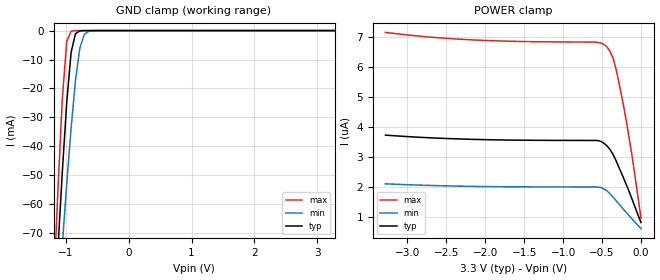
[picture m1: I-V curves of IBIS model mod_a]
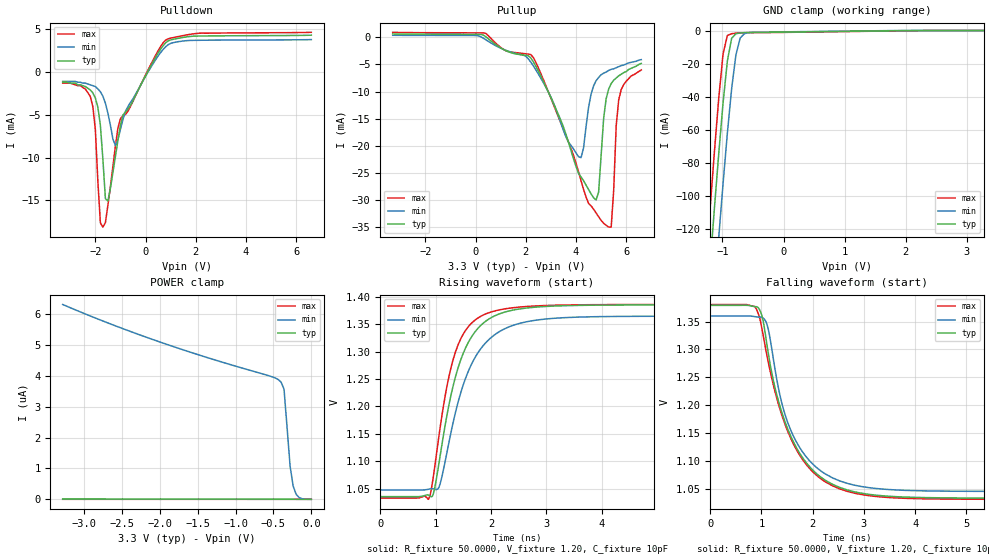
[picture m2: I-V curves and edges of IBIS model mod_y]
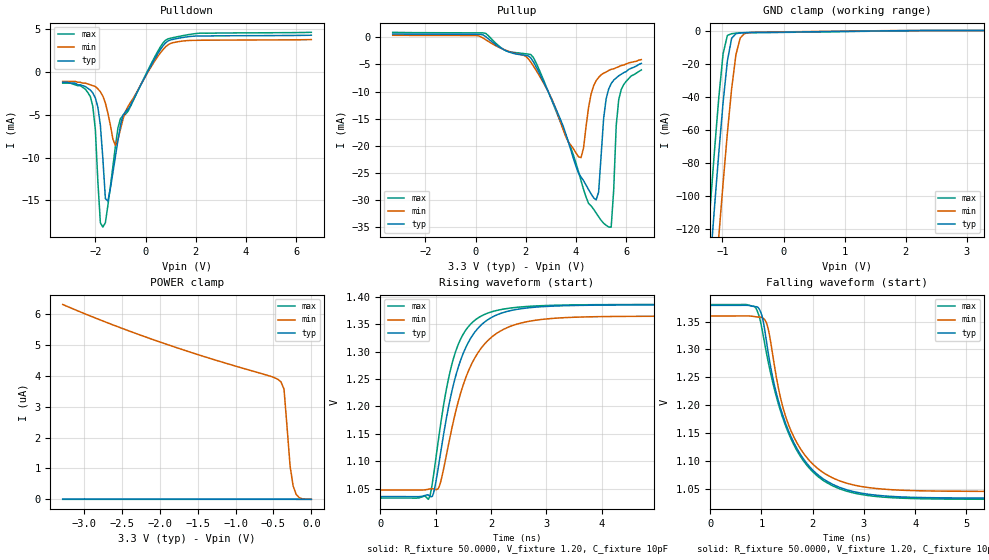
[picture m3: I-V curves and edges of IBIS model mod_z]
| IBIS (I/O, Buffer, Information, Specification) Model, officially
| electronic behavioral standard for Buffer structures of digital pins.
[IBIS ver]  4.0
[File name] rhflvds31a_3v3_rev3.ibs
[File Rev]  1.0
[Date]   28 Apr 2021
[Source]   CAD & Design Services (Catania) - STMicroelectronics
[Notes]
   (Note1)  This IBIS model is the model of the product with package
   (Flat16 package elements);
   (Note2)  This IBIS model is extracted with nominal 3.3V power supply
   (min:3.0V, typ:3.3V, max:3.6V);
   (Note3)  This IBIS model has some Notes about the non-monotonicity
   of the I-V curves, but they are not indicative of problems
   inside the model;
[Disclaimer] Customers are solely responsible for all aspects of their
   own product designs or applications using this IBIS Model.
   STMicroelectronics assumes no liability for Custmer
   Designs and applications associated to this IBIS Model.
   In the use of this IBIS Model Customer shall not modify,
   disassemble, alter this Model in whole or in part.
   If Customers do not accept these terms, the IBIS Model
   may not be used. For any problems or modifications please
   contact STMicroelectronics (www.st.com).
[Copyright] (c) 2021 STMicroelectronics
|   Component RHFLVDS31A
[Component] RHFLVDS31A
[Manufacturer] STMicroelectronics
[Package]
| variable   typ   min   max
R_pkg   0.0   0.0   0.0
L_pkg   0.0H   0.0H   0.0H
C_pkg   0.0F   0.0F   0.0F
[Pin]   signal_name   model_name   R_pin   L_pin   C_pin
1   1A   mod_a   0.0   0.0   0.0
2   1Y   mod_y   0.0   0.0   0.0
3   1Z   mod_z   0.0   0.0   0.0
4   G   mod_g   0.0   0.0   0.0
5   2Z   mod_z   0.0   0.0   0.0
6   2Y   mod_y   0.0   0.0   0.0
7   2A   mod_a   0.0   0.0   0.0
8   GND   GND   0.0   0.0   0.0
9   3A   mod_a   0.0   0.0   0.0
10   3Y   mod_y   0.0   0.0   0.0
11   3Z   mod_z   0.0   0.0   0.0
12   GN   mod_g   0.0   0.0   0.0
13   4Z   mod_z   0.0   0.0   0.0
14   4Y   mod_y   0.0   0.0   0.0
15   4A   mod_a   0.0   0.0   0.0
16   VCC   POWER   0.0   0.0   0.0
[Diff pin]  inv_pin   vdiff   tdelay_typ  tdelay_min  tdelay_max
2   3   0V   0.0s   0.0s   0.0s
6   5   0V   0.0s   0.0s   0.0s
10   11   0V   0.0s   0.0s   0.0s
14   13   0V   0.0s   0.0s   0.0s
[Package Model]  292448_RHFLVDS31_IBIS
[Define Package Model]  292448_RHFLVDS31_IBIS
[Manufacturer]  STMicroelectronics
[OEM]  STMicroelectronics
[Description]  ceramic flat-16
[Number Of Pins]  16
[Pin Numbers]
|Pin Num   Terminal Name
1   | NET1:bw1_source
2   | NET2:bw2_source
3   | NET3:bw3_source
4   | NET4:bw4_source
5   | NET5:bw5_source
6   | NET6:bw6_source
7   | NET7:bw7_source
8   | NET8:bw8_source
9   | NET9:bw9_source
10   | NET10:bw10_source
11   | NET11:bw11_source
12   | NET12:bw12_source
13   | NET13:bw13_source
14   | NET14:bw14_source
15   | NET15:bw15_source
16   | NET16:bw16_source
[Model Data]
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[End Model Data]
[End Package Model]
| Models and submodels in the file (4): mod_a (Input), mod_y (3-state), mod_z (3-state), mod_g (Input)
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|   Model mod_a
[Model]   mod_a
Model_type Input
Vinl   =   0.6500V
Vinh   =   1.2000V
C_comp   0.075pF   0.072pF   0.079pF
[Temperature Range]  25.0000   0.1250k   -55.0000
[Voltage Range]   3.3000V   3.0000V   3.6000V
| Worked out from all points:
|   GND clamp passes 1 mA (typ) near -0.85 V on its own axis
[GND_clamp]
|Voltage   I(typ)   I(min)   I(max)
-3.3V     -1.037A    -847.3mA   -1.291A
-1.2V     -103.9mA   -118.4mA   -90.61mA
-1.13V    -75.7mA    -95.97mA   -55.15mA
-1.06V    -48.92mA   -74.09mA   -23.64mA
-990mV    -24.98mA   -53.14mA   -3.768mA
-920mV    -7.585mA   -33.75mA   -179.6uA
-850mV    -1.057mA   -17.22mA   -5.053uA
-780mV    -97.1uA    -5.969mA   -122.7nA
-710mV    -6.82uA    -1.339mA   -2.974nA
-640mV    -449.9nA   -233.7uA   -80.51pA
-500mV    -1.943nA   -4.459uA   -7.043pA
3.28V     3.538uA    1.987uA    6.819uA
[POWER_clamp]
|Voltage   I(typ)   I(min)   I(max)
-3.28V    3.717uA    2.092uA    7.145uA
-2.24V    3.582uA    2.011uA    6.906uA
-560mV    3.539uA    1.988uA    6.813uA
-480mV    3.455uA    1.928uA    6.753uA
-440mV    3.369uA    1.867uA    6.673uA
-400mV    3.249uA    1.766uA    6.522uA
-360mV    3.079uA    1.654uA    6.302uA
-320mV    2.869uA    1.533uA    5.922uA
-240mV    2.389uA    1.289uA    4.922uA
-200mV    2.138uA    1.169uA    4.362uA
-120mV    1.618uA    937nA      3.121uA
0V        803nA      596.8nA    940.7nA
|   Model mod_y
[Model]   mod_y
Model_type 3-state
|Vinl   =   0.99V
|Vinh   =   1.26V
Polarity   Non-Inverting
Enable   Active-High
Vmeas  =   1.650V
Cref   =   10pF
C_comp   0.321pF   0.255pF   0.355pF
[Temperature Range]   25.0000   0.1250k   -55.0000
[Voltage Range]   3.3000V   3.0000V   3.6000V
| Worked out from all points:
|   slope of the pulldown table from 0 to 0.495 V, typ, clamps not added: 189 ohm
|   slope of the pullup table from 0 to 0.495 V, typ, clamps not added: 636 ohm
|   GND clamp passes 1 mA (typ) near -0.04 V on its own axis
|   rising waveform, R_fixture 50.0000, V_fixture 1.20, C_fixture 10pF: 20-80 % time 508ps typ, 593ps min, 416ps max; typ from 1.03 V to 1.39 V
|   falling waveform, R_fixture 50.0000, V_fixture 1.20, C_fixture 10pF: 20-80 % time 725ps typ, 659ps min, 752ps max; typ from 1.38 V to 1.03 V
[Pulldown]
|Voltage   I(typ)   I(min)   I(max)
-3.3V     -1.2mA     -1.1mA     -1.3mA
-2.2V     -2.1mA     -1.5mA     -2.87mA
-2V       -3.04mA    -1.7mA     -6.72mA
-1.9V     -4.11mA    -1.97mA    -12.77mA
-1.8V     -6.22mA    -2.31mA    -17.61mA
-1.7V     -10.17mA   -2.82mA    -18.12mA
-1.6V     -14.79mA   -3.64mA    -17.59mA
-1.5V     -15.07mA   -4.82mA    -15.56mA
-1.2V     -9.84mA    -8.59mA    -8.63mA
-900mV    -5.024mA   -5.524mA   -5.101mA
800mV     3.413mA    2.947mA    3.726mA
6.6V      4.296mA    3.783mA    4.632mA
[Pullup]
|Voltage   I(typ)   I(min)   I(max)
-3.3V     647.6uA    399.4uA    947.4uA
100mV     579.3uA    314.7uA    847.9uA
2.2V      -3.796mA   -4.572mA   -3.171mA
4.2V      -25.81mA   -22.22mA   -26.5mA
4.8V      -30.05mA   -8mA       -32.46mA
4.9V      -28.59mA   -7.39mA    -33.16mA
5.1V      -14.94mA   -6.6mA     -34.36mA
5.3V      -9.54mA    -6.1mA     -35.06mA
5.4V      -8.53mA    -5.9mA     -35.08mA
5.6V      -7.5mA     -5.6mA     -16.31mA
5.7V      -7.1mA     -5.4mA     -11.52mA
6.6V      -4.8mA     -4.1mA     -6mA
[GND_clamp]
|Voltage   I(typ)   I(min)   I(max)
-3.3V     -1.345A    -1.575A    -1.253A
-1.27V    -175.3mA   -229.2mA   -141.4mA
-1.2V     -140.6mA   -192.8mA   -106.4mA
-1.13V    -106.6mA   -158.1mA   -72.36mA
-1.06V    -73.96mA   -124.6mA   -40.43mA
-990mV    -43.62mA   -92.45mA   -14.06mA
-920mV    -18.43mA   -62.15mA   -2.993mA
-850mV    -4.705mA   -35.21mA   -1.919mA
-780mV    -1.922mA   -14.74mA   -1.598mA
-710mV    -1.49mA    -4.531mA   -1.403mA
-640mV    -1.316mA   -1.864mA   -1.318mA
3.28V     23.54pA    1.078uA    19.83pA
[POWER_clamp]
|Voltage   I(typ)   I(min)   I(max)
-3.28V    10.31nA    6.317uA    198.2pA
-2.68V    8.946nA    5.716uA    177.1pA
-2.04V    7.686nA    5.138uA    154.7pA
-560mV    5.402nA    4.006uA    102.7pA
-440mV    5.247nA    3.889uA    98.42pA
-400mV    5.194nA    3.807uA    96.77pA
-360mV    5.137nA    3.571uA    94.08pA
-280mV    4.92nA     1.078uA    85.8pA
-240mV    4.209nA    433.6nA    68.63pA
-200mV    1.594nA    161nA      33.42pA
-160mV    407.8pA    56.33nA    25.64pA
0V        24.13pA    1.061nA    22.9pA
[Ramp]
| variable   typ   min   max
dV/dt_r   0.4405/0.4439n   0.3885/0.4693n   0.4915/0.4754n
dV/dt_f   0.4405/0.2435n   0.3885/0.2716n   0.4915/0.2233n
R_load = 50.0000
[Rising Waveform]
R_fixture= 50.0000   |   New Rising 10pF
V_fixture= 1.20
V_fixture_min= 1.20
V_fixture_max= 1.20
C_fixture = 10pF
|time   V(typ)   V(min)   V(max)
0s        1.035V     1.047V     1.033V
870ps     1.038V     1.049V     1.03V
940ps     1.036V     1.05V      1.059V
1.08ns    1.109V     1.058V     1.16V
1.22ns    1.192V     1.124V     1.245V
1.36ns    1.255V     1.19V      1.3V
1.64ns    1.326V     1.275V     1.351V
1.98ns    1.361V     1.324V     1.372V
3.38ns    1.384V     1.362V     1.385V
10ns      1.385V     1.365V     1.386V
[Falling Waveform]
R_fixture= 50.0000   |  New Falling 10pF
V_fixture= 1.20
V_fixture_min= 1.20
V_fixture_max= 1.20
C_fixture = 10pF
|time   V(typ)   V(min)   V(max)
0s        1.379V     1.36V      1.381V
860ps     1.377V     1.359V     1.378V
1.05ns    1.342V     1.355V     1.317V
1.13ns    1.295V     1.337V     1.278V
1.29ns    1.222V     1.251V     1.215V
1.61ns    1.137V     1.147V     1.133V
1.99ns    1.084V     1.095V     1.081V
2.53ns    1.052V     1.064V     1.049V
3.93ns    1.034V     1.046V     1.032V
10ns      1.033V     1.045V     1.031V
|   Model mod_z
[Model]   mod_z
Model_type 3-state
|Vinl   =   0.99V
|Vinh   =   1.26V
Polarity   Inverting
Enable   Active-Low
Vmeas  =   1.650V
Cref   =   10pF
C_comp   0.321pF   0.255pF   0.355pF
[Temperature Range]   25.0000   0.1250k   -55.0000
[Voltage Range]   3.3000V   3.0000V   3.6000V
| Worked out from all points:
|   slope of the pulldown table from 0 to 0.495 V, typ, clamps not added: 189 ohm
|   slope of the pullup table from 0 to 0.495 V, typ, clamps not added: 636 ohm
|   GND clamp passes 1 mA (typ) near -0.04 V on its own axis
|   rising waveform, R_fixture 50.0000, V_fixture 1.20, C_fixture 10pF: 20-80 % time 508ps typ, 593ps min, 416ps max; typ from 1.03 V to 1.39 V
|   falling waveform, R_fixture 50.0000, V_fixture 1.20, C_fixture 10pF: 20-80 % time 725ps typ, 659ps min, 752ps max; typ from 1.38 V to 1.03 V
[Pulldown]
|Voltage   I(typ)   I(min)   I(max)
-3.3V     -1.2mA     -1.1mA     -1.3mA
-2.2V     -2.1mA     -1.5mA     -2.87mA
-2V       -3.04mA    -1.7mA     -6.72mA
-1.9V     -4.11mA    -1.97mA    -12.77mA
-1.8V     -6.22mA    -2.31mA    -17.61mA
-1.7V     -10.17mA   -2.82mA    -18.12mA
-1.6V     -14.79mA   -3.64mA    -17.59mA
-1.5V     -15.07mA   -4.82mA    -15.56mA
-1.2V     -9.84mA    -8.59mA    -8.63mA
-900mV    -5.024mA   -5.524mA   -5.101mA
800mV     3.413mA    2.947mA    3.726mA
6.6V      4.296mA    3.783mA    4.632mA
[Pullup]
|Voltage   I(typ)   I(min)   I(max)
-3.3V     647.6uA    399.4uA    947.4uA
100mV     579.3uA    314.7uA    847.9uA
2.2V      -3.796mA   -4.572mA   -3.171mA
4.2V      -25.81mA   -22.22mA   -26.5mA
4.8V      -30.05mA   -8mA       -32.46mA
4.9V      -28.59mA   -7.39mA    -33.16mA
5.1V      -14.94mA   -6.6mA     -34.36mA
5.3V      -9.54mA    -6.1mA     -35.06mA
5.4V      -8.53mA    -5.9mA     -35.08mA
5.6V      -7.5mA     -5.6mA     -16.31mA
5.7V      -7.1mA     -5.4mA     -11.52mA
6.6V      -4.8mA     -4.1mA     -6mA
[GND_clamp]
|Voltage   I(typ)   I(min)   I(max)
-3.3V     -1.345A    -1.575A    -1.253A
-1.27V    -175.3mA   -229.2mA   -141.4mA
-1.2V     -140.6mA   -192.8mA   -106.4mA
-1.13V    -106.6mA   -158.1mA   -72.36mA
-1.06V    -73.96mA   -124.6mA   -40.43mA
-990mV    -43.62mA   -92.45mA   -14.06mA
-920mV    -18.43mA   -62.15mA   -2.993mA
-850mV    -4.705mA   -35.21mA   -1.919mA
-780mV    -1.922mA   -14.74mA   -1.598mA
-710mV    -1.49mA    -4.531mA   -1.403mA
-640mV    -1.316mA   -1.864mA   -1.318mA
3.28V     23.54pA    1.078uA    19.83pA
[POWER_clamp]
|Voltage   I(typ)   I(min)   I(max)
-3.28V    10.31nA    6.317uA    198.2pA
-2.68V    8.946nA    5.716uA    177.1pA
-2.04V    7.686nA    5.138uA    154.7pA
-560mV    5.402nA    4.006uA    102.7pA
-440mV    5.247nA    3.889uA    98.42pA
-400mV    5.194nA    3.807uA    96.77pA
-360mV    5.137nA    3.571uA    94.08pA
-280mV    4.92nA     1.078uA    85.8pA
-240mV    4.209nA    433.6nA    68.63pA
-200mV    1.594nA    161nA      33.42pA
-160mV    407.8pA    56.33nA    25.64pA
0V        24.13pA    1.061nA    22.9pA
[Ramp]
| variable   typ   min   max
dV/dt_r   0.4405/0.4439n   0.3885/0.4693n   0.4915/0.4754n
dV/dt_f   0.4405/0.2435n   0.3885/0.2716n   0.4915/0.2233n
R_load = 50.0000
[Rising Waveform]
R_fixture= 50.0000   |   New Rising 10pF
V_fixture= 1.20
V_fixture_min= 1.20
V_fixture_max= 1.20
C_fixture = 10pF
|time   V(typ)   V(min)   V(max)
0s        1.035V     1.047V     1.033V
870ps     1.038V     1.049V     1.03V
940ps     1.036V     1.05V      1.059V
1.08ns    1.109V     1.058V     1.16V
1.22ns    1.192V     1.124V     1.245V
1.36ns    1.255V     1.19V      1.3V
1.64ns    1.326V     1.275V     1.351V
1.98ns    1.361V     1.324V     1.372V
3.38ns    1.384V     1.362V     1.385V
10ns      1.385V     1.365V     1.386V
[Falling Waveform]
R_fixture= 50.0000   |  New Falling 10pF
V_fixture= 1.20
V_fixture_min= 1.20
V_fixture_max= 1.20
C_fixture = 10pF
|time   V(typ)   V(min)   V(max)
0s        1.379V     1.36V      1.381V
860ps     1.377V     1.359V     1.378V
1.05ns    1.342V     1.355V     1.317V
1.13ns    1.295V     1.337V     1.278V
1.29ns    1.222V     1.251V     1.215V
1.61ns    1.137V     1.147V     1.133V
1.99ns    1.084V     1.095V     1.081V
2.53ns    1.052V     1.064V     1.049V
3.93ns    1.034V     1.046V     1.032V
10ns      1.033V     1.045V     1.031V
